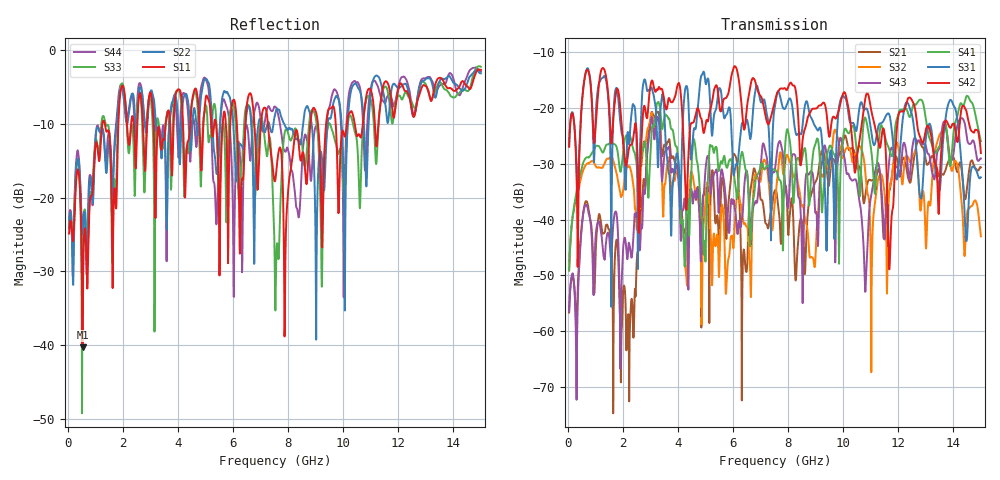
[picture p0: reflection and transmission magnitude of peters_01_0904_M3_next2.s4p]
# MHZ S RI R 50.00
! FREQ  S11  S12  S13  S14
!  S21  S22  S23  S24
!  S31  S32  S33  S34
!  S41  S42  S43  S44
!  REAL  IMAG  REAL  IMAG  REAL  IMAG  REAL  IMAG
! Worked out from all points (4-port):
!   1496 points, 50 MHz to 15 GHz, reference 50 ohm
!   strongest paths, dB at 50 MHz, 3.79 GHz, 7.53 GHz, 11.27 GHz, 15 GHz:
!     S42: -27.0, -19.0, -18.7, -25.9, -28.1
!     S31: -26.9, -35.8, -19.5, -23.5, -32.5
!     S41: -49.1, -23.8, -31.1, -27.2, -26.0
!     S43: -56.4, -31.1, -30.8, -29.9, -29.1
!     S32: -49.1, -33.8, -36.5, -32.8, -43.0
!     S21: -56.6, -28.9, -34.7, -31.1, -30.7
!   lowest |S11| = -40.3 dB at 540 MHz (marker M1), VSWR 1.02, Z = 50.8 + j0.51 ohm
!   |S11| at or under -10 dB: start of sweep to 1.257 GHz; 1.345 GHz to 1.84 GHz (494.6 MHz wide, 31.1 % of centre); 7.265 GHz to 8.808 GHz (1.543 GHz wide, 19.2 % of centre)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
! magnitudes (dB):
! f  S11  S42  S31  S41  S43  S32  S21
! 50 MHz  -24.9  -27.0  -26.9  -49.1  -56.4  -49.1  -56.6
! 540 MHz  -40.3  -17.7  -17.7  -30.2  -39.9  -31.5  -39.6
! 2.19 GHz  -12.1  -28.3  -24.4  -24.8  -45.8  -30.5  -57.3
! 3.07 GHz  -7.3  -15.2  -16.9  -23.4  -22.0  -21.1  -20.9
! 4.28 GHz  -18.0  -35.5  -16.3  -43.3  -37.9  -49.1  -42.8
! 6.37 GHz  -17.5  -23.0  -22.9  -28.6  -37.6  -40.2  -46.2
! 15 GHz  -2.7  -28.1  -32.5  -26.0  -29.1  -43.0  -30.7
